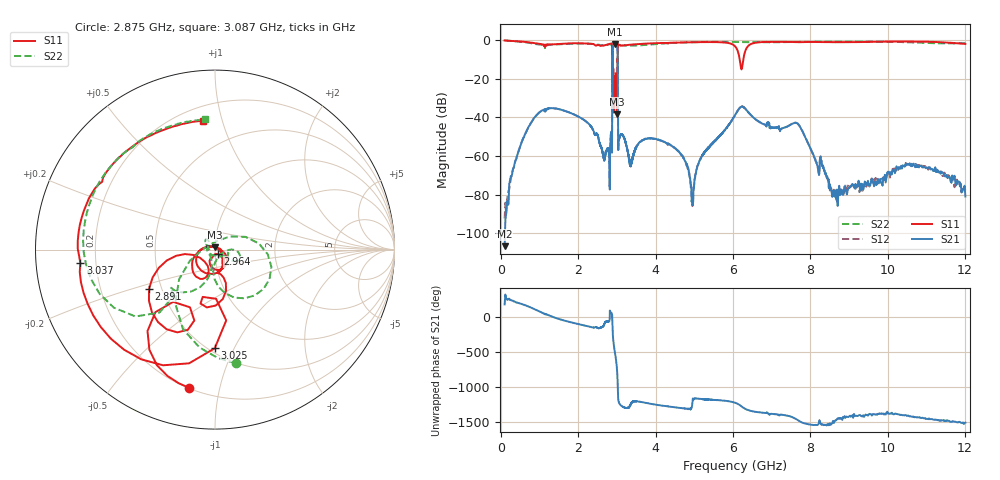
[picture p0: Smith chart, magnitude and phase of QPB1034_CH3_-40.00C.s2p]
! TDS: k:\Engsetup\Winsaw\QPB1034_ALL
! Channel 1
! Ports=1 2
! seg 1=100.000000 1100.000000 51
! seg 2=1101.000000 1301.000000 201
! seg 3=1302.000000 2302.000000 101
! seg 4=2303.000000 3503.000000 1201
! seg 5=3504.000000 5204.000000 171
! seg 6=5205.000000 6405.000000 1201
! seg 7=6406.000000 8506.000000 211
! seg 8=8507.000000 12007.000000 176
! Points=3313
! FailCode=0
! Topology=ALL_SE(12)
!VNA Cal loaded =QPB1034_ALL_-40C
!PS1(V)= 5.000
!PS(mA)= 0.424
!PS2(V)= 0.630
!PS(mA)= -0.001
!PS3(V)= 1.170
!PS(mA)= 0.000
!PS4(V)= 1.170
!PS(mA)= -0.001
!Temp (C)= -40.00
# MHz S DB R 50
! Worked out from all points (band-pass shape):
!   3313 points, 100 MHz to 12.01 GHz, reference 50 ohm
!   highest |S21| = -2.22 dB at 2.952 GHz (marker M1); lowest = -106.6 dB at 100 MHz (marker M2)
!   |S21| within 3 dB of the highest: 2.893 GHz to 3.018 GHz (124.6 MHz wide, 4.21 % of centre)
!   lowest |S11| = -38.4 dB at 3 GHz (marker M3), VSWR 1.02, Z = 49.8 + j1.18 ohm
!   |S11| at or under -10 dB: 2.893 GHz to 3.019 GHz (126.1 MHz wide, 4.27 % of centre); 3.020647 GHz to 3.023379 GHz (2.732 MHz wide, 0.0904 % of centre); 6.175 GHz to 6.268 GHz (92.87 MHz wide, 1.49 % of centre)
!   |S22| runs from -30.1 to -0.3 dB; largest |S21 - S12| = 0.005
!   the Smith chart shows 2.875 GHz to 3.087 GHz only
!   S11 on the Smith chart (normalised r, x): 2.875 GHz: 0.20, -0.81; 2.891 GHz: 0.43, -0.23; 2.964 GHz: 1.03, -0.05; 3.025 GHz: 0.53, -0.84; 3.037 GHz: 0.14, -0.05; 3.087 GHz: 0.29, +0.87
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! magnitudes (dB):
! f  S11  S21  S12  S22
! 100 MHz  -0.3  -106.6  -92.3  -0.3
! 240 MHz  -0.4  -72.5  -74.1  -0.5
! 500 MHz  -0.8  -55.1  -55.2  -0.9
! 1.1 GHz  -2.3  -36.1  -36.1  -2.6
! 2.434 GHz  -2.6  -48.8  -48.7  -2.5
! 2.811 GHz  -2.1  -65.8  -66.5  -2.3
! 2.875 GHz  -2.1  -56.9  -57.2  -3.8
! 2.891 GHz  -7.4  -6.5  -6.5  -9.4
! 2.952 GHz  -22.4  -2.2  -2.2  -27.6
! 2.964 GHz  -30.9  -2.4  -2.4  -29.9
! 3 GHz  -38.4  -3.0  -3.0  -26.3
! 3.025 GHz  -5.2  -15.7  -15.7  -4.7
! 3.037 GHz  -2.4  -55.6  -55.6  -2.5
! 3.087 GHz  -2.8  -49.6  -49.6  -2.7
! 3.352 GHz  -2.5  -64.4  -64.1  -2.9
! 4.944 GHz  -1.2  -81.2  -82.8  -1.2
! 5.406 GHz  -1.1  -54.8  -54.8  -1.0
! 6.251 GHz  -12.3  -34.5  -34.5  -1.1
! 7.676 GHz  -1.2  -43.3  -43.3  -1.0
! 8.647 GHz  -1.2  -77.7  -79.9  -0.8
! 10.67 GHz  -0.8  -63.9  -65.1  -1.3
! 12.01 GHz  -2.0  -80.9  -78.0  -1.7
